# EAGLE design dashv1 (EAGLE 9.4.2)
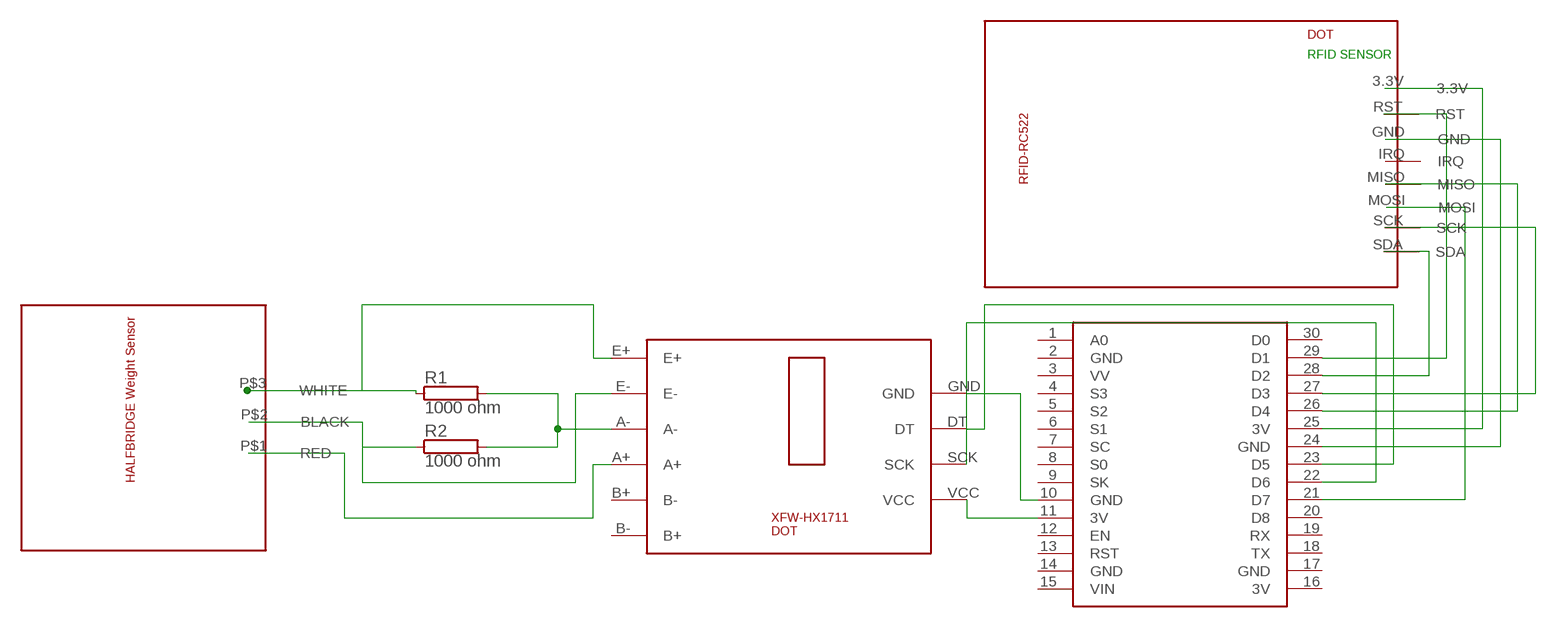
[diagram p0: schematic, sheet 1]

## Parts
R1  1000 ohm  RAC03  [AC03]
R2  1000 ohm  RAC03  [AC03]
U$1  NODEMCU  [NODEMCU]
U$2  HX1711  [HX711]
U$3  RFIDCUSTOM  [RFIDCUSTOM]
U$4  HALFBRIDGE  [HALFBRIDGE]

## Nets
N$1: R1.1 U$2.E+ U$4.P$3(WHITE)
N$2: R1.2 R2.2 U$2.A-
N$3: R2.1 U$2.E- U$4.P$2(BLACK)
N$4: U$2.A+ U$4.P$1(RED)
N$5: U$1.10(GND) U$2.GND
N$6: U$1.11(3V) U$2.VCC
N$7: U$1.23(D5) U$2.DT
N$8: U$1.22(D6) U$2.SCK
N$9: U$1.25(3V) U$3.3.3V
N$10: U$1.24(GND) U$3.GND
N$11: U$1.29(D1) U$3.RST
N$12: U$1.21(D7) U$3.MOSI
N$13: U$1.28(D2) U$3.SDA
N$14: U$1.26(D4) U$3.MISO
N$15: U$1.27(D3) U$3.SCK
Unconnected: U$1.1(A0) U$1.3(VV) U$1.4(S3) U$1.5(S2) U$1.6(S1) U$1.7(SC) U$1.8(S0) U$1.9(SK) U$1.12(EN) U$1.13(RST) U$1.15(VIN) U$1.18(TX) U$1.19(RX) U$1.20(D8) U$1.30(D0) U$2.B+(B-) U$2.B-(B+) U$3.IRQ

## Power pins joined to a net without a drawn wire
3V: U$1.16(3V)
GND: U$1.2(GND) U$1.14(GND) U$1.17(GND)

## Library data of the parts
R1 R2 = resistor-power:R: Power Resitor; OC_FARNELL: unknown; OC_NEWARK: unknown
U$1 = nodemcu:NODEMCU
U$2 = hx1711custom:HX1711
U$3 = RFID Custom:RFIDCUSTOM
U$4 = HalfBridge:HALFBRIDGE

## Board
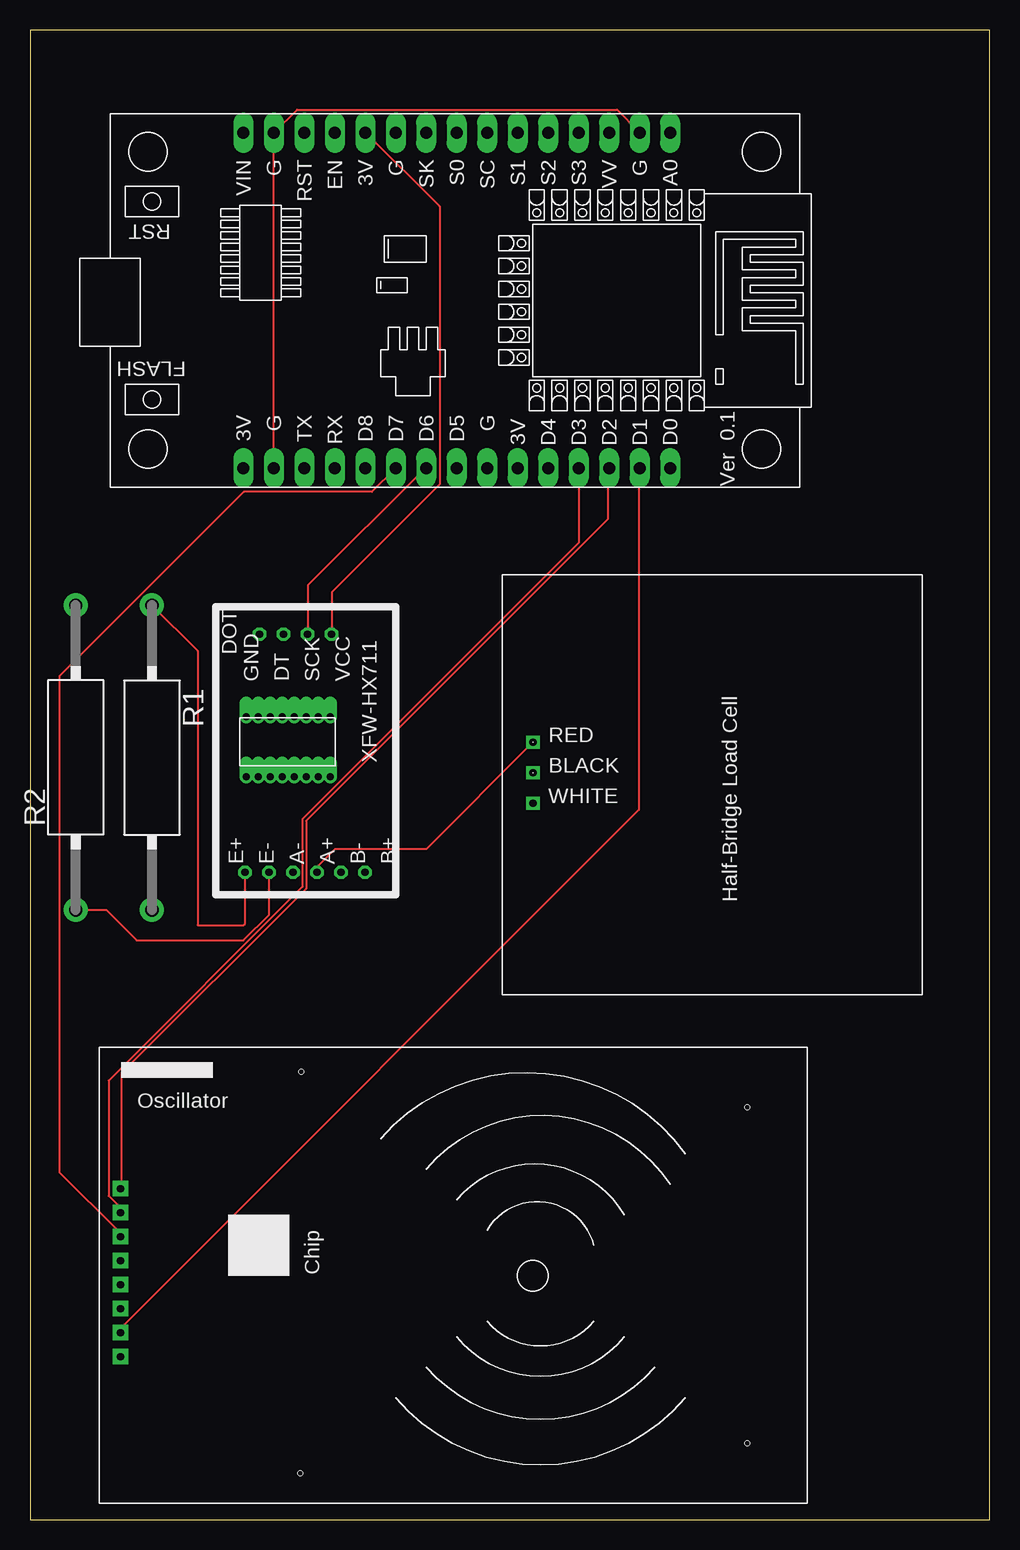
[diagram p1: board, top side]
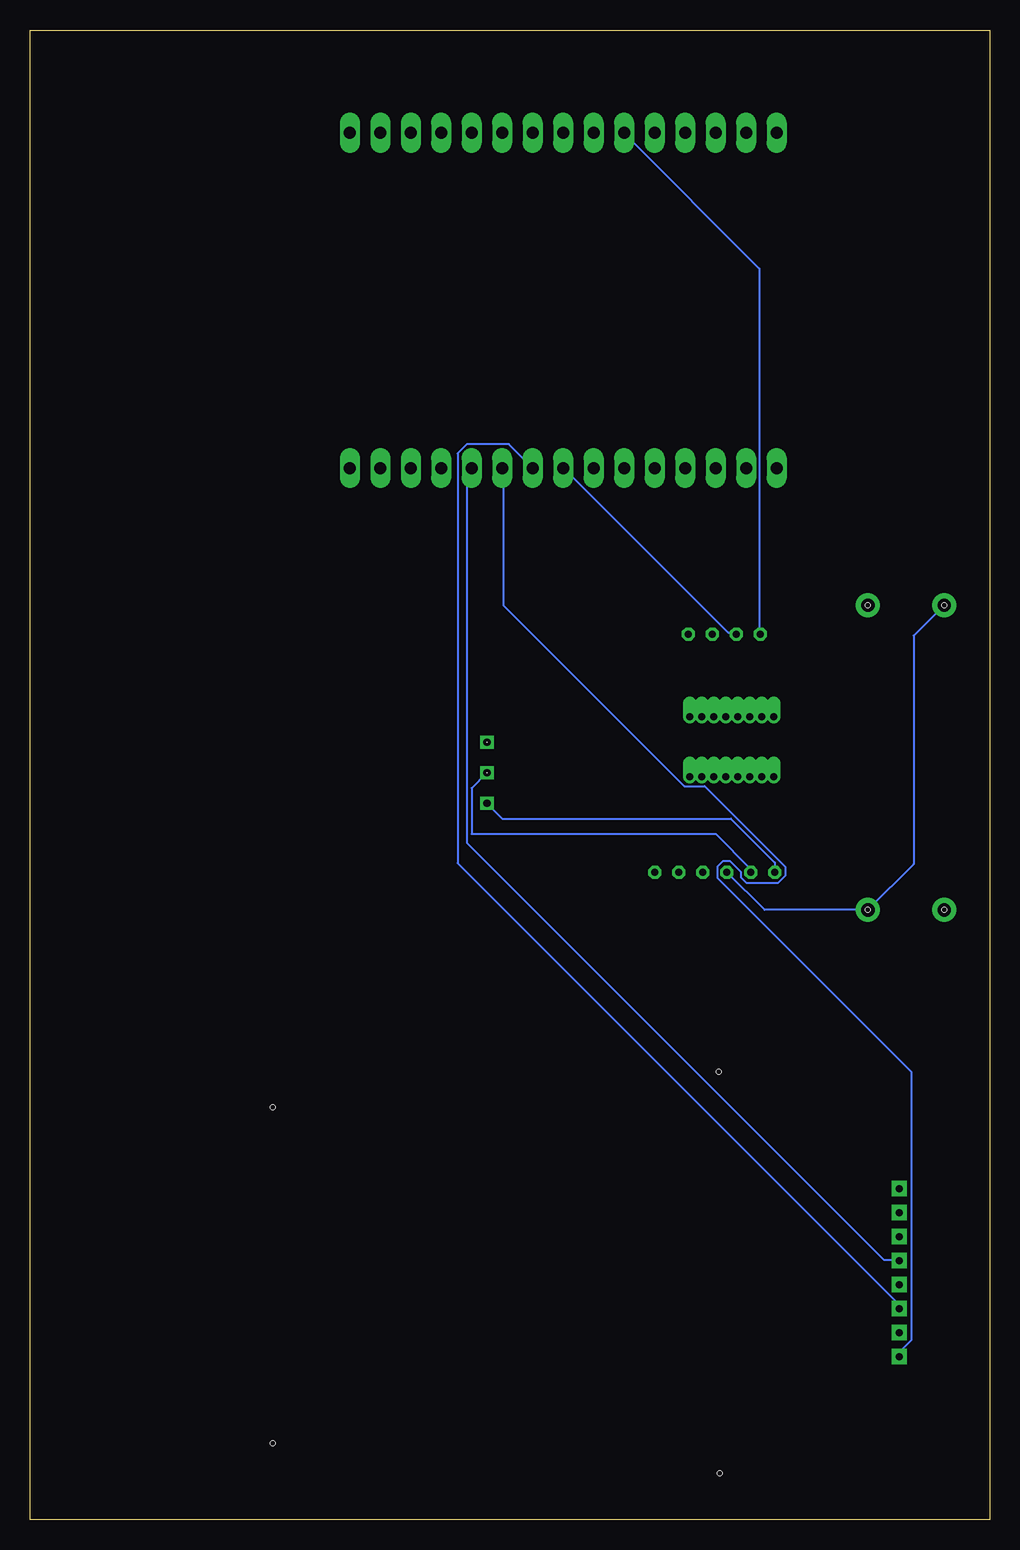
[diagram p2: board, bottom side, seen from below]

Size 79.99 x 124.13 mm. Coordinates in mm from the lower left corner, seen from the top.
Outline: 0,0 79.99,0 79.99,124.13 0,124.13 0,0
Copper layers (1*16): Top 0.035mm / dielectric 1.5mm / Bottom 0.035mm
Design rules "default": minimum track width 6mil, minimum drill 0.35mm, track to track 6mil, track to pad 6mil, pad to pad 6mil, via to via 6mil, smd to smd 6mil, copper to edge 40mil, drill to drill 6mil, minimum pad ring 10mil, minimum via ring 8mil, stop-mask expansion 4mil, vias tented up to drill 0mil, thermal gap 10mil
Holes 0.4 mm at 10.16,76.2 3.81,76.2 3.81,50.8 10.16,50.8
Holes 0 mm at 41.91,64.77 41.91,62.23

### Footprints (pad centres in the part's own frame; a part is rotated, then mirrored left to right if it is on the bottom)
AC03 = drill 1.1 pad 2: 1 -12.7,0; 2 12.7,0
NODEMCU = drill 1 pad 1.676 long: 1 -13.97,17.78; 2 -13.97,15.24; 3 -13.97,12.7; 4 -13.97,10.16; 5 -13.97,7.62; 6 -13.97,5.08; 7 -13.97,2.54; 8 -13.97,0; 9 -13.97,-2.54; 10 -13.97,-5.08; 11 -13.97,-7.62; 12 -13.97,-10.16; 13 -13.97,-12.7; 14 -13.97,-15.24; 15 -13.97,-17.78; 16 13.97,-17.78; 17 13.97,-15.24; 18 13.97,-12.7; 19 13.97,-10.16; 20 13.97,-7.62; 21 13.97,-5.08; 22 13.97,-2.54; 23 13.97,0; 24 13.97,2.54; 25 13.97,5.08; 26 13.97,7.62; 27 13.97,10.16; 28 13.97,12.7; 29 13.97,15.24; 30 13.97,17.78
HX711 = drill 0.6 octagon: A+ 1.87,6.56; A- 1.87,8.56; B+ 1.87,2.56; B- 1.87,4.56; DT 21.71,9.35; E+ 1.87,12.56; E- 1.87,10.56; GND 21.71,11.35; SCK 21.71,7.35; VCC 21.71,5.35 | drill 0.6 offset: S0 9.84,12.47; S1 9.84,11.47; S2 9.84,10.47; S3 9.84,9.47; S4 9.84,8.47; S5 9.84,7.47; S6 9.84,6.47; S7 9.84,5.47; S8 14.84,5.47; S9 14.84,6.47; S10 14.84,7.47; S11 14.84,8.47; S12 14.84,9.47; S13 14.84,10.47; S14 14.84,11.47; S15 14.84,12.47
RFIDCUSTOM = drill 0.6 pad 1.27 square: 3.3V 57.22,25.79; GND 57.22,21.79; IRQ 57.22,19.79; MISO 57.22,17.79; MOSI 57.22,15.79; RST 57.22,23.79; SCK 57.22,13.79; SDA 57.22,11.79 | hole 0.4: 5,33; 5,5; 42.26,35.5; 42.18,2.06
HALFBRIDGE = drill 0.6 square: P$1 13.97,2.54; P$2 16.51,2.54; P$3 19.05,2.54

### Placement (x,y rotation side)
R1  10.16,63.5 270 top
R2  3.81,63.5 90 top
U$1  35.56,101.6 270 top
U$2  30.48,52.07 90 top
U$3  64.77,39.37 180 top
U$4  39.37,78.74 270 top

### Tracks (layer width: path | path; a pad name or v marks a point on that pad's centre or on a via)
GND
  Top 0.152: U$1.17 20.27,87.63 20.27,115.52 U$1.14 22.25,117.5 48.92,117.5 50.75,115.67 U$1.2
N$1
  Top 0.152: R1.1 13.97,72.39 13.97,49.53 17.78,49.53 17.92,49.67 U$2.E+
  Bottom 0.152: U$4.P$3 40.64,58.42 21.59,58.42 17.92,54.75 U$2.E+
N$2
  Bottom 0.152: U$2.A- 18.78,50.8 R1.2 6.35,54.61 6.35,73.66 R2.2
N$3
  Top 0.152: R2.1 6.35,50.8 8.89,48.26 17.78,48.26 19.92,50.4 U$2.E-
  Bottom 0.152: U$4.P$2 43.18,60.96 43.18,57.15 22.86,57.15 19.92,54.21 U$2.E-
N$4
  Top 0.152: U$4.P$1 33.02,55.88 25.4,55.88 23.92,54.4 U$2.A+
N$5
  Bottom 0.152: U$2.GND 19.2,73.91 19.2,104.24 30.48,115.52 U$1.10
N$6
  Top 0.152: U$2.VCC 25.15,73.91 25.15,77.27 34.14,86.26 34.14,109.42 28.04,115.52 U$1.11
N$7
  Bottom 0.152: U$2.DT 21.18,73.91 21.79,73.91 35.51,87.63 U$1.23
N$8
  Top 0.152: U$2.SCK 23.16,73.91 23.16,77.88 32.92,87.63 U$1.22
N$9
  Bottom 0.152: U$3.3.3V 7.47,13.72 7.47,14.02 6.55,14.94 6.55,37.34 22.71,53.49 22.71,54.41 22.25,54.86 21.64,54.86 20.73,53.95 20.73,53.49 20.27,53.03 17.68,53.03 17.07,53.65 17.07,54.41 23.77,61.11 25.45,61.11 40.54,76.2 40.54,87.63 U$1.25
N$10
  Bottom 0.152: U$1.24 40.08,89.61 43.59,89.61 44.35,88.85 44.35,54.71 7.62,17.98 7.62,17.68 U$3.GND
N$11
  Top 0.152: U$3.RST 7.62,15.7 7.62,16 50.75,59.13 50.75,87.63 U$1.29
N$12
  Top 0.152: U$1.21 28.5,85.65 17.83,85.65 2.44,70.26 2.44,28.96 7.47,23.93 7.47,23.62 U$3.MOSI
N$13
  Top 0.152: U$3.SDA 7.62,27.58 7.62,37.19 23.01,52.58 23.01,58.22 48.16,83.36 48.16,87.63 U$1.28
N$14
  Bottom 0.152: U$3.MISO 7.62,21.64 8.84,21.64 43.59,56.39 43.59,87.33 43.28,87.63 U$1.26
N$15
  Top 0.152: U$1.27 45.72,81.38 22.71,58.37 22.71,52.73 6.55,36.58 6.55,26.98 7.47,26.06 7.47,25.6 U$3.SCK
